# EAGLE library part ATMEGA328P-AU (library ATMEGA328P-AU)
ATmega Series 20 MHz 32 KB Flash 2 KB SRAM 8-Bit Microcontroller - TQFP-32
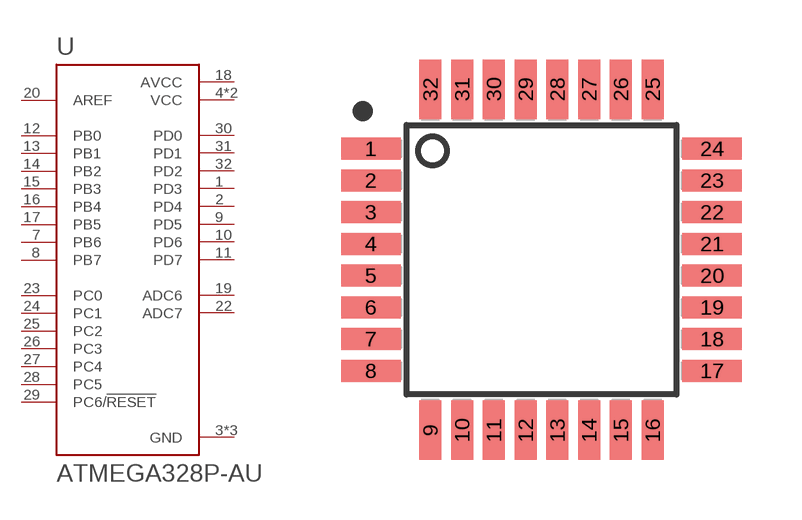
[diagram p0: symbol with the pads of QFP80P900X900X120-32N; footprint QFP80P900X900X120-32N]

Designator prefix U

## ATMEGA328P-AU (Availability: Unavailable; Description: Microcontroller Mcu, 8 Bit, Atmega, 20mhz, Tqfp-32; MF: Microchip; MP: ATMEGA328P-AU; Package: TQFP-32 Microchip; Price: None)  [QFP80P900X900X120-32N]
1  PD3
2  PD4
3  GND  pwr
4  VCC  pwr
5  GND  pwr
6  VCC  pwr
7  PB6
8  PB7
9  PD5
10  PD6
11  PD7
12  PB0
13  PB1
14  PB2
15  PB3
16  PB4
17  PB5
18  AVCC  pwr
19  ADC6
20  AREF  in
21  GND  pwr
22  ADC7
23  PC0
24  PC1
25  PC2
26  PC3
27  PC4
28  PC5
29  PC6/!RESET
30  PD0
31  PD1
32  PD2

## Footprint QFP80P900X900X120-32N (pad centres in mm)
smd 1.5 x 0.55: 1 -4.3,2.8; 2 -4.3,2; 3 -4.3,1.2; 4 -4.3,0.4; 5 -4.3,-0.4; 6 -4.3,-1.2; 7 -4.3,-2; 8 -4.3,-2.8; 17 4.3,-2.8; 18 4.3,-2; 19 4.3,-1.2; 20 4.3,-0.4; 21 4.3,0.4; 22 4.3,1.2; 23 4.3,2; 24 4.3,2.8
smd 0.55 x 1.5: 9 -2.8,-4.3; 10 -2,-4.3; 11 -1.2,-4.3; 12 -0.4,-4.3; 13 0.4,-4.3; 14 1.2,-4.3; 15 2,-4.3; 16 2.8,-4.3; 25 2.8,4.3; 26 2,4.3; 27 1.2,4.3; 28 0.4,4.3; 29 -0.4,4.3; 30 -1.2,4.3; 31 -2,4.3; 32 -2.8,4.3

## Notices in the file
This work is licensed under a Creative Commons Attribution-ShareAlike 4.0 International License (CC BY-SA) with Design Exception 1.0
